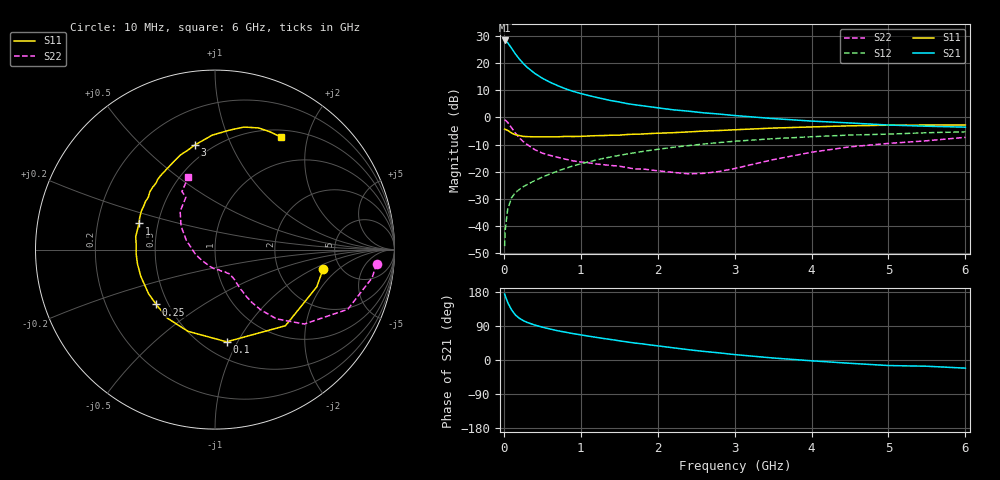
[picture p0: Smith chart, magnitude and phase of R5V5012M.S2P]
! SIEMENS Small Signal Semiconductors
! BFR183
! Si NPN RF Bipolar Junction Transistor in SOT23
! VCE = 0.5 V  IC = 12 mA
! Common Emitter S-Parameters:  May  1996
# GHz  S  MA  R  50
!  f  S11  S21  S12  S22
! GHz  MAG  ANG  MAG  ANG  MAG  ANG  MAG  ANG
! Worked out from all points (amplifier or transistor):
!   36 points, 10 MHz to 6 GHz, reference 50 ohm
!   highest |S21| = 28.3 dB at 10 MHz (marker M1)
!   |S21| within 3 dB of that: start of sweep to 104 MHz
!   unconditionally stable (mu >= 1): 460 MHz to 4.333 GHz; 4.722 GHz to end of sweep
!   at 250 MHz: K = 0.76, MSG = 22.7 dB, |S12| = -25.5 dB
!   at 1.4 GHz: K = 1.14, MAG = 8.1 dB, |S12| = -14.5 dB
!   at 6 GHz: K = 1.02, MAG = 0.1 dB, |S12| = -5.3 dB
!   S11 on the Smith chart (normalised r, x): 10 MHz: 3.70, -1.26; 100 MHz: 0.64, -0.90; 250 MHz: 0.43, -0.33; 1 GHz: 0.39, +0.14; 3 GHz: 0.41, +0.74; 6 GHz: 0.59, +1.58
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0.01  0.6122 -10.0  26 174.2  0.0043 83.9  0.9041 -5.1
0.02  0.6038 -20.1  25.81 167.9  0.0089 80.5  0.8892 -10.2
0.05  0.578 -47.2  23.7 151.9  0.0206 70.4  0.8114 -24.2
0.1  0.5178 -82.8  18.78 132.4  0.0334 60.3  0.6476 -39.8
0.15  0.4796 -108.3  14.71 118.8  0.0415 55.4  0.516 -48.4
0.2  0.4652 -124.8  11.93 110.4  0.0472 54.7  0.4233 -52.7
0.25  0.4479 -137.0  9.909 104.2  0.053 54.4  0.3619 -55.0
0.3  0.4443 -146.3  8.415 99.4  0.0582 55.4  0.3192 -56.1
0.4  0.4395 -160.2  6.488 92.4  0.0687 57.7  0.2571 -57.1
0.5  0.4392 -169.4  5.261 86.7  0.08 58.9  0.2206 -57.2
0.6  0.4402 -177.2  4.441 81.8  0.0913 59.9  0.201 -57.0
0.7  0.4404 175.9  3.84 77.2  0.1034 60.4  0.1847 -57.4
0.8  0.4477 170.7  3.371 73.4  0.1158 60.2  0.1713 -58.3
1  0.4485 161.0  2.751 66.4  0.1404 59.8  0.1517 -60.5
1.1  0.4559 157.0  2.534 63.0  0.1523 59.3  0.1465 -63.1
1.6  0.4854 138.4  1.799 47.7  0.2126 54.5  0.1201 -76.4
2.2  0.5243 120.5  1.381 32.2  0.2824 46.9  0.0979 -107.5
3  0.593 101.1  1.084 14.3  0.3649 35.4  0.115 -170.4
3.5  0.6377 91.4  0.953 5.3  0.4065 28.0  0.1674 162.2
4.5  0.7015 76.7  0.791 -8.7  0.4746 14.5  0.2884 132.3
5.5  0.7244 64.8  0.689 -16.5  0.5237 3.3  0.3727 119.6
6  0.7265 59.8  0.663 -21.5  0.5436 -3.9  0.4307 110.1
